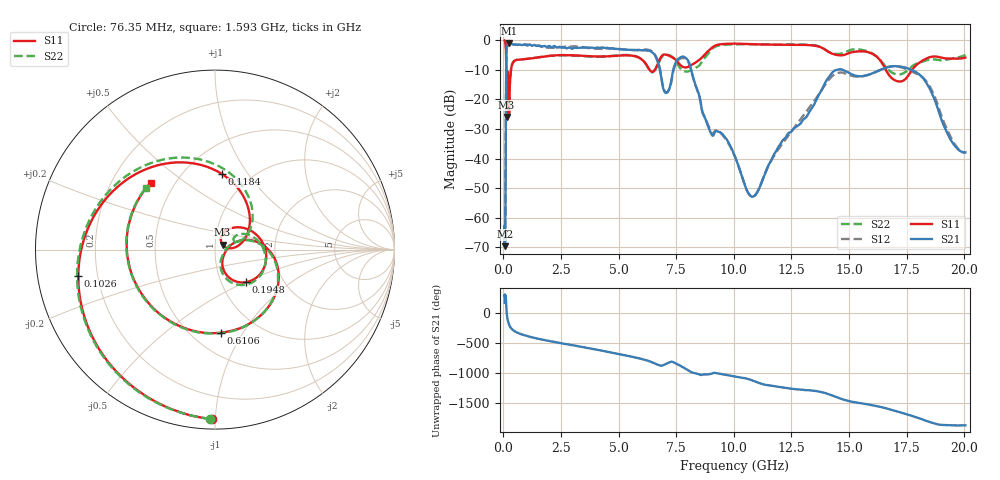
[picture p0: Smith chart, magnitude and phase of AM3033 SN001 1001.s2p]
# Hz S DB R 50
!freq MagS11 AngS11 MagS21 AngS21 MagS12 AngS12 MagS22 AngS22
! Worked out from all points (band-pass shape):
!   1601 points, 50 MHz to 20.05 GHz, reference 50 ohm
!   highest |S21| = -0.95 dB at 257 MHz (marker M1); lowest = -69.6 dB at 68.75 MHz (marker M2)
!   |S21| within 3 dB of the highest: 130.5 MHz to 6.423 GHz (6.292 GHz wide, 192 % of centre)
!   lowest |S11| = -25.9 dB at 134.9 MHz (marker M3), VSWR 1.11, Z = 54.3 + j3.09 ohm
!   |S11| at or under -10 dB: 121.6 MHz to 328.2 MHz (206.7 MHz wide, 91.9 % of centre); 6.337 GHz to 6.572 GHz (235.2 MHz wide, 3.64 % of centre); 16.59 GHz to 17.74 GHz (1.153 GHz wide, 6.72 % of centre)
!   |S22| runs from -25.7 to -0.1 dB; largest |S21 - S12| = 0.063
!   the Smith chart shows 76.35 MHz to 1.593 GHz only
!   S11 on the Smith chart (normalised r, x): 76.35 MHz: 0.06, -0.98; 102.6 MHz: 0.13, -0.09; 118.4 MHz: 0.75, +0.77; 194.8 MHz: 1.30, -0.50; 610.6 MHz: 0.69, -0.81; 1.593 GHz: 0.37, +0.37
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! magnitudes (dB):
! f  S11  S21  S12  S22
! 50 MHz  -0.1  -62.9  -68.9  -0.1
! 68.75 MHz  -0.3  -69.6  -65.3  -0.4
! 76.35 MHz  -0.5  -65.4  -65.5  -0.5
! 102.6 MHz  -2.2  -29.8  -29.8  -2.2
! 118.4 MHz  -7.5  -9.7  -9.7  -6.9
! 134.9 MHz  -25.9  -3.3  -3.3  -18.7
! 135.9 MHz  -25.8  -3.2  -3.2  -18.7
! 156.7 MHz  -12.4  -2.3  -2.3  -11.9
! 194.8 MHz  -12.1  -1.5  -1.5  -12.2
! 238.5 MHz  -24.5  -1.0  -1.0  -25.5
! 257 MHz  -20.6  -1.0  -1.0  -20.7
! 369.6 MHz  -8.4  -1.4  -1.3  -8.4
! 610.6 MHz  -6.7  -1.6  -1.6  -6.6
! 1.005 GHz  -6.4  -1.8  -1.5  -6.4
! 1.593 GHz  -5.7  -1.9  -2.2  -5.7
! 2.722 GHz  -5.1  -2.8  -2.4  -5.1
! 7.402 GHz  -6.2  -9.1  -9.6  -6.2
! 7.978 GHz  -9.1  -6.5  -6.9  -10.6
! 10.77 GHz  -1.4  -52.8  -52.8  -1.4
! 14.58 GHz  -5.1  -9.9  -11.0  -4.7
! 17.78 GHz  -9.6  -10.3  -10.9  -8.6
! 20.05 GHz  -5.9  -37.9  -38.0  -5.0
